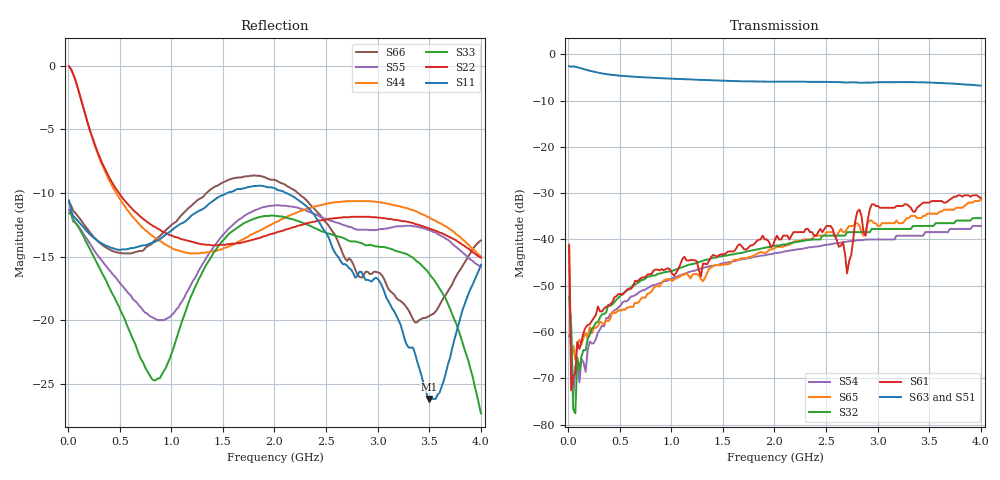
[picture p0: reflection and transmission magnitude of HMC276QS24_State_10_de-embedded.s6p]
! Hittite Microwave Corporation
! 20 Alpha Road
! Chelmsford, MA 01824
! Tel: 978-250-3343
! Fax: 978-250-3373
! Device: HMC276QS24, 0.7-3.0 GHz, GaAS MMIC 4x2 Switch Matrix in 24-lead QSOP package
! Misc: Data was de-embedded to package pins.
!  Port 1 = OP1
!  Port 2 = VL
!  Port 3 = VH
!  Port 4 = HH
!  Port 5 = HL
!  Port 6 = OP2
!  Vdd = +5 V
!  Vctl = 0 V[Logic 0] / +5 V[Logic 1]
!  State 10,  HL to OP1,  VH to OP2
!  Control Lines (Logic)
!  HV 1 = 1, Tone 1 = 0
!  HV 2 = 0, Tone 2 = 1
!  Data reformated to new Touchstone file format - Wed Jan 10 15:51:44 2007
# MHz S DB R 50
! 6 Port Network Data
! freq  dbS11  angS11  dbS12  angS12  dbS13  angS13  dbS14  angS14
!  dbS15  angS15  dbS16  angS16
!  dbS21  angS21  dbS22  angS22
!  dbS23  angS23  dbS24  angS24  dbS25  angS25  dbS26  angS26
!  dbS31  angS31  dbS32  angS32  dbS33  angS33  dbS34  angS34
!  dbS35  angS35  dbS36  angS36
!  dbS41  angS41  dbS42  angS42
!  dbS43  angS43  dbS44  angS44  dbS45  angS45  dbS46  angS46
!  dbS51  angS51  dbS52  angS52  dbS53  angS53  dbS54  angS54
!  dbS55  angS55  dbS56  angS56
!  dbS61  angS61  dbS62  angS62
!  dbS63  angS63  dbS64  angS64  dbS65  angS65  dbS66  angS66
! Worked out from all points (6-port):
!   201 points, 10 MHz to 4 GHz, reference 50 ohm
!   strongest paths, dB at 10 MHz, 1.008 GHz, 2.005 GHz, 3.002 GHz, 4 GHz:
!     S63: -2.6, -5.3, -5.9, -6.0, -6.8
!     S51: -2.8, -5.3, -6.0, -6.2, -6.9
!     S61: -41.3, -47.4, -40.0, -32.8, -31.1
!     S32: -52.4, -46.8, -41.4, -37.7, -35.4
!     S65: -41.1, -48.9, -41.8, -37.1, -31.4
!     S54: -60.9, -48.4, -42.9, -40.0, -37.1
!   lowest |S11| = -26.2 dB at 3.501 GHz (marker M1), VSWR 1.10, Z = 50.4 + j4.91 ohm
!   |S11| at or under -10 dB: start of sweep to 1.541 GHz; 2.112 GHz to end of sweep
